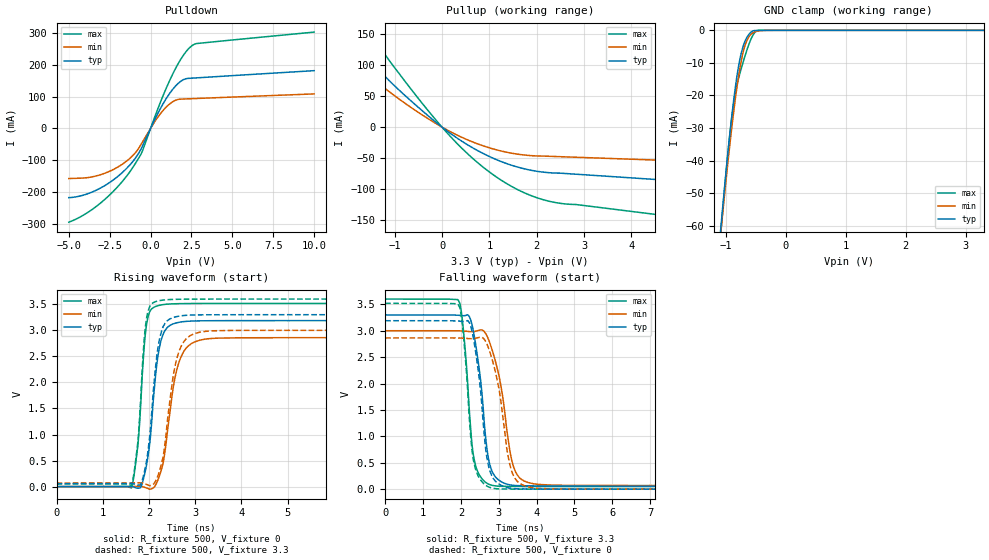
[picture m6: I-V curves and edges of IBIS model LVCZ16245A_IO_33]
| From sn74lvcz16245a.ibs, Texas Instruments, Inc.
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[Model]   LVCZ16245A_IO_33
Model_type  I/O
Vinl = 0.8
Vinh = 2
Enable   Active-Low
Vref =   0
Rref =   500
Cref =   50p
Vmeas =   1.65
| variable   typ   min   max
C_comp   3.48pF   2.91pF   4.13pF
| C_pullup   4.61pF   3.97pF   5.12pF
| C_pulldown   5.75pF   2.95pF   8.16pF
| C_tri-state   3.48pF   2.91pF   4.13pF
[Temperature Range]   40   100   -40
| Ambient temperature   25   85   -40
[Voltage range]   3.3   3   3.6
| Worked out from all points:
|   slope of the pulldown table from 0 to 0.495 V, typ, clamps not added: 9.48 ohm
|   slope of the pullup table from 0 to 0.495 V, typ, clamps not added: 18.8 ohm
|   GND clamp passes 1 mA (typ) near -0.60 V on its own axis
|   rising waveform, R_fixture 500, V_fixture 0: 20-80 % time 215ps typ, 286ps min, 161ps max; typ from 0 V to 3.19 V
|   falling waveform, R_fixture 500, V_fixture 3.3: 20-80 % time 291ps typ, 396ps min, 226ps max; typ from 3.3 V to 0.058 V
|   rising waveform, R_fixture 500, V_fixture 3.3: 20-80 % time 211ps typ, 270ps min, 156ps max; typ from 0.058 V to 3.3 V
|   falling waveform, R_fixture 500, V_fixture 0: 20-80 % time 279ps typ, 374ps min, 221ps max; typ from 3.19 V to 0 V
[GND Clamp]
| LVCZ16245A_IO_33
|   Voltage   I(typ)   I(min)   I(max)
-5V       -1.044A    -987.9mA   -1.125A
-1.085V   -60.91mA   -62.35mA   -62.41mA
-1.06V    -55.83mA   -57.62mA   -56.91mA
-975mV    -39.36mA   -42.2mA    -39.41mA
-910mV    -27.91mA   -31.31mA   -28.08mA
-855mV    -19.37mA   -22.93mA   -20.76mA
-805mV    -12.9mA    -16.19mA   -16.06mA
-750mV    -7.532mA   -10.05mA   -12.18mA
-695mV    -4.021mA   -5.561mA   -8.748mA
-565mV    -355.5uA   -977uA     -2.077mA
-465mV    -20.7uA    -218.9uA   -16.1uA
3.3V      1.121nA    115.6nA    -203.4pA
[Pulldown]
| LVCZ16245A_IO_33
|   Voltage   I(typ)   I(min)   I(max)
-5V       -218.1mA   -158mA     -295.4mA
-4.045V   -209.2mA   -156.1mA   -271.3mA
-3.05V    -187.5mA   -145.7mA   -234.7mA
-2.075V   -154.2mA   -123.9mA   -187.3mA
-1.23V    -113mA     -92.7mA    -133.9mA
-520mV    -58.33mA   -45.13mA   -73.84mA
345mV     37.13mA    27.98mA    48.29mA
995mV     96.93mA    69.12mA    131mA
1.79V     146.1mA    92mA       212.9mA
2.505V    158.1mA    93.52mA    259.4mA
2.845V    159.2mA    94.22mA    267.5mA
10V       181.8mA    108.6mA    303.3mA
[Pullup]
| LVCZ16245A_IO_33
|   Voltage   I(typ)   I(min)   I(max)
-5V       413.7mA    329.4mA    576.4mA
-2.765V   212mA      165.7mA    299.3mA
-2.2V     163.8mA    127.1mA    232.5mA
-1.625V   116.4mA    89.43mA    166.1mA
-1.57V    112mA      85.91mA    159.7mA
-715mV    46.42mA    34.91mA    67.25mA
-90mV     5.435mA    4.019mA    8.013mA
415mV     -22.52mA   -16.29mA   -33.74mA
1.26V     -55.8mA    -38.68mA   -86.02mA
2.125V    -72.44mA   -46.66mA   -116.7mA
6.62V     -95.08mA   -58.82mA   -160.8mA
10V       -112.3mA   -68.02mA   -193.2mA
[Ramp]
| LVCZ16245A_IO_33
| variable   typ   min   max
dV/dt_r   1.93/2.25E-10   1.74/2.95E-10   2.13/1.64E-10
dV/dt_f   1.95/2.93E-10   1.77/4.02E-10   2.13/2.33E-10
R_load = 500
[Rising Waveform]
| LVCZ16245A_IO_33
R_fixture =   500
C_fixture =   0
L_fixture =   0
V_fixture =   0
V_fixture_min = 0
V_fixture_max = 0
|   Time   V(typ)   V(min)   V(max)
0s        114.6pV    2.853nV    6.968nV
1.62ns    6.263mV    1.389mV    -27.7mV
1.76ns    -28.88mV   6.297mV    789.3mV
1.96ns    477.7mV    -30.03mV   3.171V
2.195ns   2.508V     130.9mV    3.473V
2.405ns   3.061V     1.098V     3.503V
2.56ns    3.134V     2.075V     3.51V
2.735ns   3.166V     2.566V     3.513V
3.465ns   3.185V     2.849V     3.516V
50ns      3.186V     2.859V     3.517V
[Falling Waveform]
| LVCZ16245A_IO_33
R_fixture =   500
C_fixture =   0
L_fixture =   0
V_fixture =   3.3
V_fixture_min = 3
V_fixture_max = 3.6
|   Time   V(typ)   V(min)   V(max)
0s        3.3V       3V         3.6V
1.94ns    3.293V     2.998V     3.565V
2.06ns    3.285V     2.995V     3.063V
2.345ns   2.933V     2.985V     585.4mV
2.515ns   2.096V     3.016V     238.7mV
2.71ns    657.7mV    2.867V     103.5mV
2.935ns   214.7mV    2.36V      59.83mV
3.395ns   71.81mV    417.2mV    51.58mV
4.065ns   60.33mV    89.2mV     50.08mV
50ns      58.1mV     68.64mV    49.54mV
[Rising Waveform]
| LVCZ16245A_IO_33
R_fixture =   500
C_fixture =   0
L_fixture =   0
V_fixture =   3.3
V_fixture_min = 3
V_fixture_max = 3.6
|   Time   V(typ)   V(min)   V(max)
0s        58.07mV    68.56mV    49.53mV
1.62ns    64.11mV    69.92mV    22.41mV
1.76ns    29.65mV    74.55mV    857.8mV
1.96ns    560.1mV    38.24mV    3.29V
2.185ns   2.604V     188.7mV    3.561V
2.36ns    3.149V     925mV      3.586V
2.535ns   3.248V     2.173V     3.594V
2.69ns    3.278V     2.679V     3.596V
3.375ns   3.299V     2.991V     3.6V
50ns      3.3V       3V         3.6V
[Falling Waveform]
| LVCZ16245A_IO_33
R_fixture =   500
C_fixture =   0
L_fixture =   0
V_fixture =   0
V_fixture_min = 0
V_fixture_max = 0
|   Time   V(typ)   V(min)   V(max)
0s        3.19V      2.864V     3.519V
1.935ns   3.184V     2.863V     3.49V
2.055ns   3.176V     2.86V      3.003V
2.255ns   3.096V     2.849V     1.038V
2.34ns    2.822V     2.851V     517.7mV
2.685ns   606.6mV    2.752V     59.71mV
2.93ns    138mV      2.164V     9.274mV
3.355ns   13.31mV    315mV      2.011mV
4.03ns    1.923mV    15.76mV    533.8uV
50ns      29.33uV    76.63uV    11.55uV
